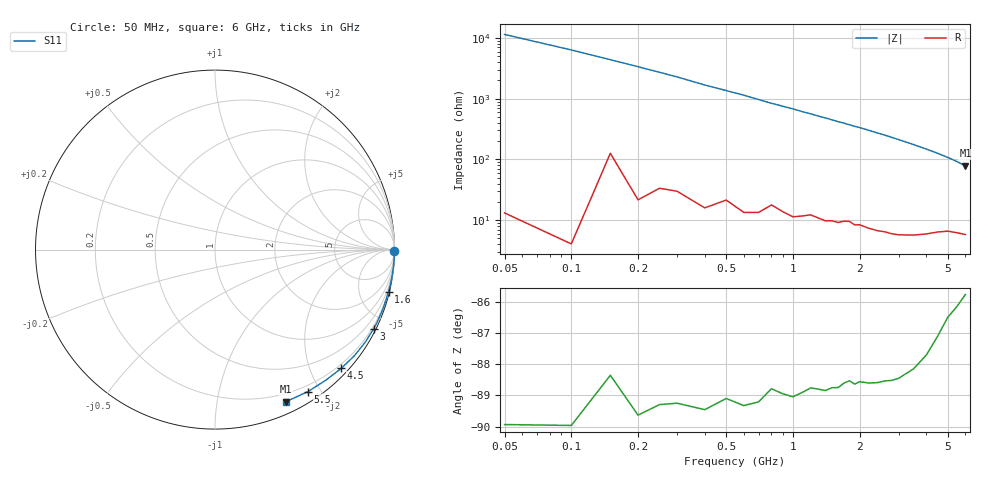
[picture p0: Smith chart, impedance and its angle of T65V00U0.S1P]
! SIEMENS Discrete & RF Semiconductors
! BAT62
! Si Schottky Diode in SOT143
! VR = 5 V
! S-Parameters:  February  1997
# GHz  S  MA  R  50
!  f  S11
! GHz  MAG  ANG
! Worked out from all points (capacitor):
!   34 points, 50 MHz to 6 GHz, reference 50 ohm
!   read as one part to ground: C = 250 fF near 50 MHz
!   lowest |Z| = 78.5 ohm at 6 GHz (marker M1)
!   S11 on the Smith chart (normalised r, x): 50 MHz: open; 1.6 GHz: 0.18, -8.38; 3 GHz: 0.11, -4.24; 4.5 GHz: 0.13, -2.52; 5.5 GHz: 0.12, -1.84; 6 GHz: 0.12, -1.57
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0.05  1 -0.5
0.15  0.9993 -1.3
0.2  0.9998 -1.7
0.3  0.9994 -2.5
0.4  0.9994 -3.4
0.6  0.999 -5.0
0.7  0.9986 -5.9
0.8  0.9975 -6.8
1  0.9976 -8.4
1.1  0.9969 -9.3
1.2  0.9962 -10.1
1.3  0.996 -11.0
1.4  0.9959 -11.8
1.6  0.9949 -13.6
1.7  0.994 -14.4
1.9  0.9934 -16.2
2  0.9927 -17.0
2.2  0.9922 -18.8
2.4  0.9914 -20.7
2.6  0.9903 -22.5
2.8  0.9893 -24.5
3  0.988 -26.5
3.5  0.9832 -31.7
4  0.976 -37.3
4.5  0.966 -43.2
5  0.9545 -49.7
5.5  0.9453 -56.8
6  0.9353 -64.9
